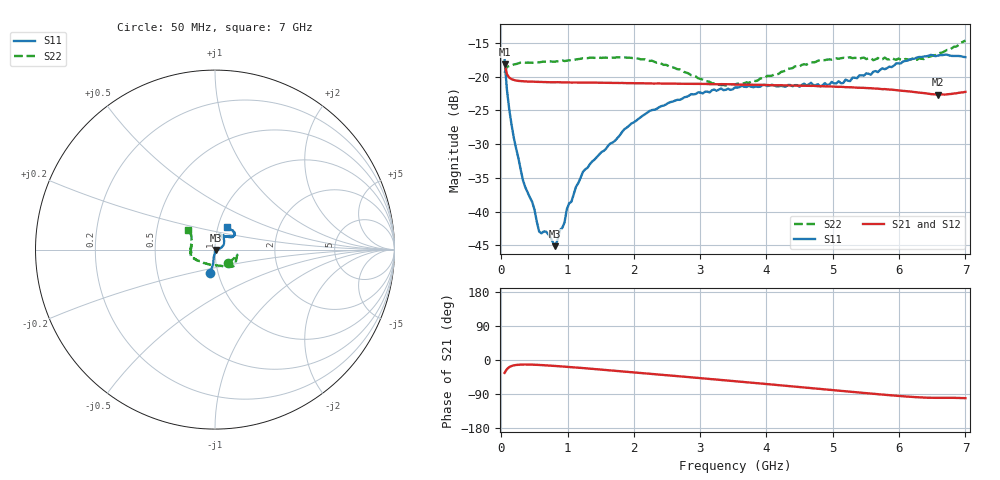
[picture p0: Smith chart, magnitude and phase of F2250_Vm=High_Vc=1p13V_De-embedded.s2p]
! Integrated Device Technology
! Corporate Headquarters
! 6024 Silver Creek Valley Road
! San Jose, CA 95138  USA
! Phone:  1-408-284-8200
! Toll Free:  1-800-223-1366
! Webpage:  http://www.idt.com/
! Timing and RF Division
! 515 Groton Road, Suite 102
! Westford, MA 01886-6024
! Device:  F2250
! Description: Voltage Variable RF Attenuator
! Frequency:  50.0 -  6000.00 MHz
! Package:  3x3 mm Thin QFN Plastic Package: 16 pin
! Ports:  2 RF, 3 DC
!  Pin  1  = GND
!  Pin  2  = NC
!  Pin  3  = RF1  = Port 1
!  Pin  4  = NC
!  Pin  5  = GND
!  Pin  6  = GND
!  Pin  7  = GND
!  Pin  8  = GND
!  Pin  9  = NC
!  Pin 10  = RF2  = Port 2
!  Pin 11  = NC
!  Pin 12  = GND
!  Pin 13  = GND
!  Pin 14  = VCNTRL
!  Pin 15  = VDD
!  Pin 16  = VMODE
! Vcntrl:  1.130 Volts
! Vmode:  +3.300 Volts
! Vdd:  +3.30  Volts
! Current:  1.329 mA
! Data:  The device was measured on a the F2250 evaluation board which has
!  individual transmission lines to the RF pins.  Data was collected
!  using a calibrated network analyzer.  The evaluation board was
!  de-embedded using a TRL calibration technique.
!  The reference plane is the edge of the package pin.
! Misc:  SN 10
!  Action Tracker AT0258
! Date Measured:  2014-11-26
! Date:  2015-10-15  MJV
! Note:
!  Integrated Device Technology supplies this data as a sample of measured
!  data at the package pin for this product.  Your particular data for this
!  product may vary.
!  Data was taken at 25 degrees C.
!  Integrated Device Technology reserves the right to change this data at anytime.
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# GHz S dB R 50
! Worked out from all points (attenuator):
!   201 points, 50 MHz to 7 GHz, reference 50 ohm
!   highest |S21| = -18.13 dB at 50 MHz (marker M1); lowest = -22.7 dB at 6.583 GHz (marker M2)
!   lowest |S11| = -45.1 dB at 814.5 MHz (marker M3), VSWR 1.01, Z = 50.5 - j0.234 ohm
!   |S11| at or under -10 dB: start of sweep to end of sweep
!   |S22| runs from -21.3 to -14.6 dB; largest |S21 - S12| = 0.00037
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0.05  -17.56 -101.9  -18.13 -33.9  -18.14 -33.9  -19.44 -45.5
0.08475  -21.92 -97.2  -19.62 -24.0  -19.63 -24.0  -18.57 -23.1
0.15425  -27.08 -99.3  -20.37 -15.9  -20.35 -15.9  -18.34 -14.1
0.328  -35.40 -92.6  -20.68 -11.9  -20.69 -11.9  -17.89 -12.9
0.467  -38.60 -90.1  -20.74 -12.2  -20.72 -12.2  -17.95 -14.8
0.57125  -42.96 -68.8  -20.77 -13.1  -20.77 -13.1  -17.88 -17.4
0.6755  -42.97 -60.0  -20.82 -14.1  -20.81 -14.1  -17.79 -19.4
0.8145  -45.13 -24.7  -20.83 -15.7  -20.82 -15.8  -17.76 -23.2
0.884  -42.73 -19.8  -20.84 -16.6  -20.83 -16.6  -17.67 -25.3
0.9535  -41.63 -26.1  -20.84 -17.5  -20.81 -17.5  -17.68 -26.6
0.98825  -39.65 -21.0  -20.84 -17.9  -20.83 -18.0  -17.64 -27.2
1.2315  -34.11 0.4  -20.87 -21.3  -20.85 -21.3  -17.25 -32.1
1.857  -27.78 20.2  -20.95 -30.4  -20.95 -30.4  -17.14 -41.3
2.37825  -24.54 33.2  -21.01 -38.2  -21.02 -38.2  -17.89 -49.6
3.1775  -22.01 55.0  -21.11 -50.6  -21.11 -50.6  -20.98 -80.4
3.525  -21.59 65.2  -21.16 -56.0  -21.17 -56.0  -21.14 -104.7
4.7065  -21.25 68.7  -21.36 -74.8  -21.38 -74.7  -17.89 -157.0
5.15825  -20.93 52.4  -21.53 -81.9  -21.53 -82.0  -17.20 -165.8
5.85325  -18.51 37.2  -21.91 -92.8  -21.91 -92.9  -17.45 179.2
6.3745  -17.01 38.7  -22.43 -99.2  -22.45 -99.2  -17.39 161.1
6.583  -16.89 42.7  -22.68 -99.8  -22.68 -99.9  -16.63 152.6
7  -17.10 61.9  -22.25 -100.7  -22.24 -100.9  -14.63 144.9
